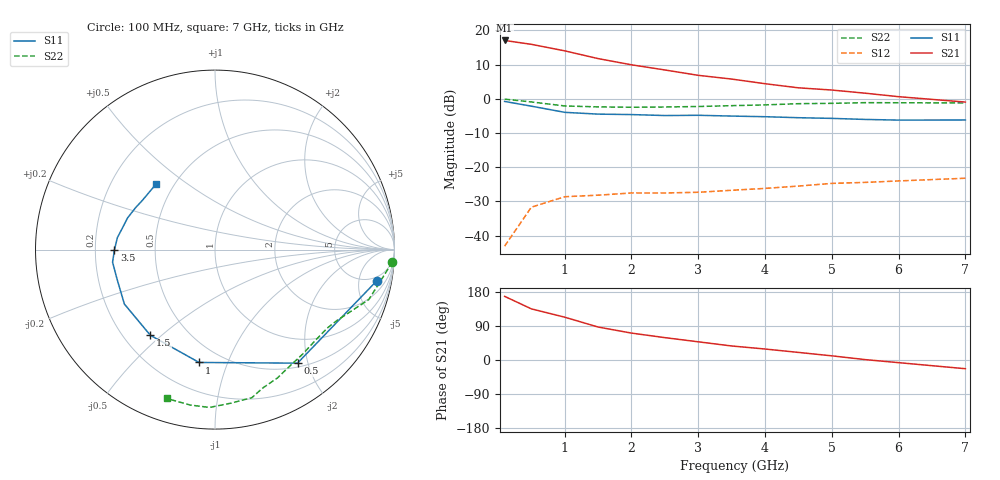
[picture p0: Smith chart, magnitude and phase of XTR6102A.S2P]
! HXTR-6102  (2N6742) Common Emitter
! Vce=10V  Ic=4mA
# ghz s ma r 50
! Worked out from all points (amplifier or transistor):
!   14 points, 100 MHz to 7 GHz, reference 50 ohm
!   highest |S21| = 17.1 dB at 100 MHz (marker M1)
!   |S21| within 3 dB of that: start of sweep to 989.2 MHz
!   unconditionally stable (mu >= 1): 2.05 GHz to 4.648 GHz; 6.169 GHz to end of sweep
!   at 1 GHz: K = 0.67, MSG = 21.3 dB, |S12| = -28.6 dB
!   at 3.5 GHz: K = 1.19, MAG = 13.6 dB, |S12| = -26.7 dB
!   at 7 GHz: K = 1.14, MAG = 8.9 dB, |S12| = -23.2 dB
!   S11 on the Smith chart (normalised r, x): 100 MHz: 3.92, -8.62; 500 MHz: 0.56, -1.83; 1 GHz: 0.38, -0.80; 1.5 GHz: 0.31, -0.46; 3.5 GHz: 0.28, +0.00; 7 GHz: 0.40, +0.38
0.1  0.917 -11.0  7.149 168.0  0.007 79.0  0.991 -4.0
0.5  0.782 -54.0  6.277 135.0  0.026 54.0  0.901 -18.0
1  0.635 -98.0  5.037 113.0  0.037 33.0  0.787 -30.0
1.5  0.598 -127.0  3.881 87.0  0.039 28.0  0.763 -35.0
2  0.589 -149.0  3.148 71.0  0.042 26.0  0.754 -43.0
2.5  0.57 -163.0  2.646 59.0  0.042 25.0  0.76 -50.0
3  0.575 -173.0  2.209 48.0  0.043 25.0  0.773 -58.0
3.5  0.56 180.0  1.948 37.0  0.046 25.0  0.795 -64.0
4  0.548 173.0  1.665 29.0  0.049 24.0  0.816 -71.0
4.5  0.53 167.0  1.45 20.0  0.053 24.0  0.85 -76.0
5  0.518 160.0  1.346 11.0  0.058 23.0  0.86 -84.0
5.5  0.5 152.0  1.21 1.0  0.06 22.0  0.88 -92.0
6  0.489 146.0  1.076 -7.0  0.063 20.0  0.877 -99.0
7  0.491 132.0  0.897 -23.0  0.069 15.0  0.872 -108.0
